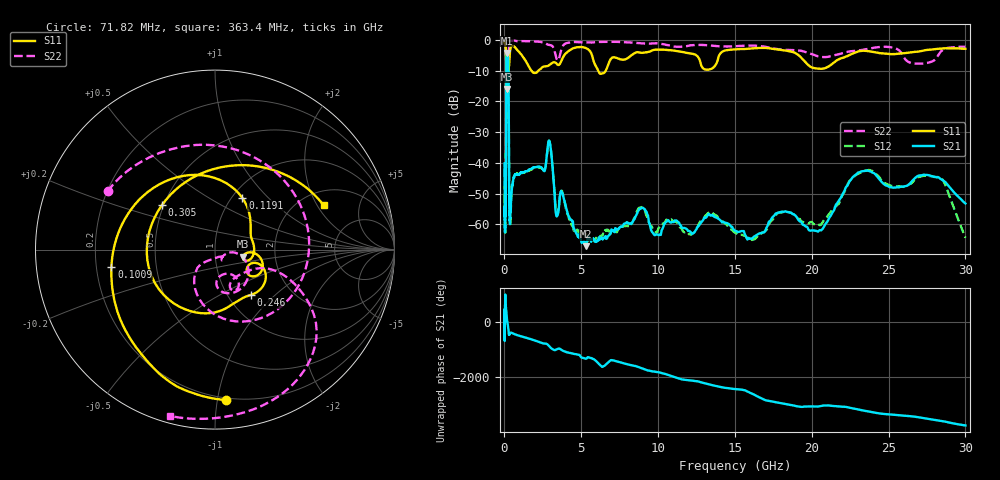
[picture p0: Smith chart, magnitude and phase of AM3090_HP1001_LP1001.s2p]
! Date/Time: Thu, Feb 28, 2019 2:03 PM
! Network Analyzer: Agilent Technologies E8364B Rev: A.07.50.67
! Sweep from 0.010 to 30.000 GHz, 1601 Points, Sweep Type: LOG
! Power Supply: 5.023 V, 0.002 A
# Hz S DB R 50
!freq MagS11 AngS11 MagS21 AngS21 MagS12 AngS12 MagS22 AngS22
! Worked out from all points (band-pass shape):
!   1601 points, 10 MHz to 30 GHz, reference 50 ohm
!   highest |S21| = -4.19 dB at 167.3 MHz (marker M1); lowest = -67.2 dB at 5.311 GHz (marker M2)
!   |S21| within 3 dB of the highest: 124.5 MHz to 252.8 MHz (128.3 MHz wide, 68 % of centre)
!   lowest |S11| = -15.9 dB at 154.4 MHz (marker M3), VSWR 1.38, Z = 68.1 - j5.53 ohm
!   |S11| at or under -10 dB: 119.5 MHz to 229.6 MHz (110.1 MHz wide, 63.1 % of centre); 1.761 GHz to 2.2 GHz (439.2 MHz wide, 22.2 % of centre); 6.102 GHz to 6.589 GHz (487.4 MHz wide, 7.68 % of centre)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
!   |S22| runs from -27.0 to -0.1 dB; largest |S21 - S12| = 0.013
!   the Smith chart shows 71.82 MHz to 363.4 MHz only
!   S11 on the Smith chart (normalised r, x): 71.82 MHz: 0.18, -1.06; 100.9 MHz: 0.26, -0.08; 119.1 MHz: 1.12, +0.72; 246 MHz: 1.27, -0.72; 305 MHz: 0.49, +0.28; 363.4 MHz: 2.64, +2.27
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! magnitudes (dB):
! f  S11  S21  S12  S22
! 10 MHz  -0.3  -40.2  -41.9  -0.7
! 38.04 MHz  -0.5  -61.5  -59.3  -1.5
! 71.82 MHz  -1.5  -52.1  -54.0  -3.3
! 84.71 MHz  -2.4  -55.2  -53.3  -4.6
! 100.9 MHz  -4.7  -34.7  -34.7  -5.5
! 119.1 MHz  -9.7  -10.3  -10.2  -13.2
! 144.7 MHz  -14.3  -4.6  -4.5  -24.7
! 154.4 MHz  -15.9  -4.3  -4.2  -21.4
! 167.3 MHz  -13.2  -4.2  -4.2  -14.2
! 246 MHz  -9.9  -6.4  -6.3  -13.2
! 270.5 MHz  -9.3  -13.6  -13.5  -9.3
! 305 MHz  -8.3  -52.3  -51.9  -1.1
! 363.4 MHz  -3.7  -59.6  -58.7  -0.4
! 550.5 MHz  -1.9  -46.2  -46.1  -0.2
! 2.084 GHz  -10.6  -41.4  -41.3  -0.5
! 2.928 GHz  -8.1  -32.9  -32.9  -1.6
! 3.402 GHz  -7.7  -57.5  -56.7  -6.3
! 5.311 GHz  -2.6  -67.2  -63.2  -0.8
! 7.926 GHz  -6.2  -59.5  -60.6  -0.7
! 20.2 GHz  -9.2  -62.1  -60.1  -4.9
! 23.48 GHz  -3.5  -42.6  -42.5  -3.0
! 30 GHz  -2.8  -53.3  -64.4  -2.2
